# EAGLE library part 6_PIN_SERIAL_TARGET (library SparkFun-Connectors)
6-pin header connection for use with the "FTDI BASIC" pinout - TARGET SIDE. Also known as "Arduino Serial Program Header". It is used to mate with our FTDI Basic serial programmers using the Arduino IDE. Note, this device has "TARGET" in the name. It is intended to be used on a design that contains a target micro-controller that you wish to program. The "sister" device, named "CABLE" is inteneded to be used on a design that usually lives on the end of your USB cable and prvides the converter chip (FTDI232 or FTDI231x) to commnicate serial RX/TX. You can populate with some of these: Break Away Headers - Straight (PRT-00116) For reference (or to suit your programming needs) check out these designs: SparkFun FTDI Basic Breakout - 5V (DEV-09716) SparkFun FTDI Basic Breakout - 3.3V (DEV-09873) SparkFun FTDI SmartBasic (DEV-12935) SparkFun Beefy 3 - FTDI Basic Breakout (DEV-13746)
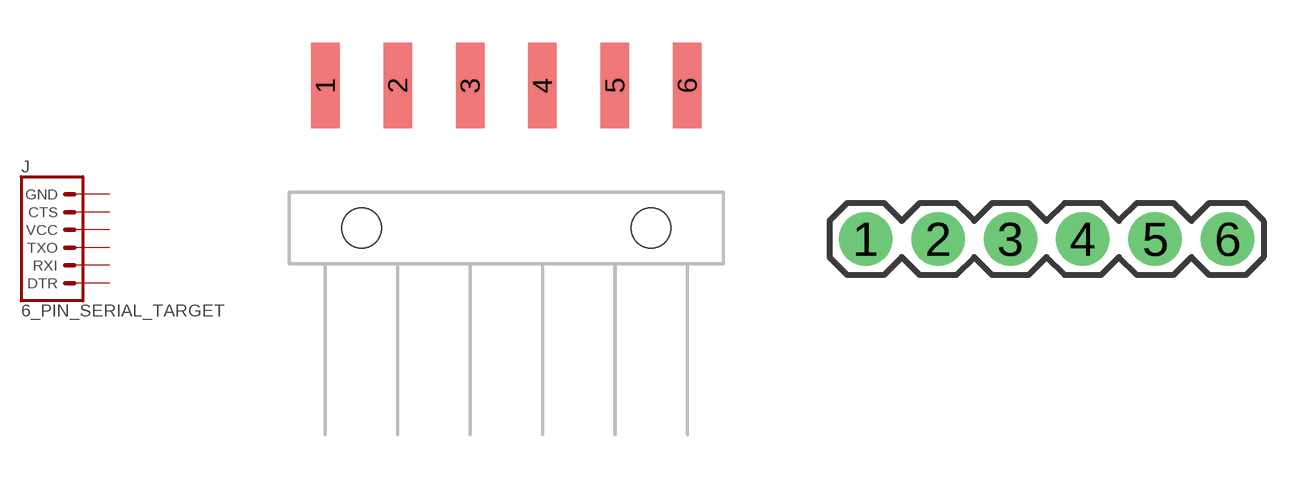
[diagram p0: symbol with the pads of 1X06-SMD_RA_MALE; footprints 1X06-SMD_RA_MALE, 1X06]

Designator prefix J

## 6_PIN_SERIAL_TARGETSMD (PROD_ID: CONN-08971)  [1X06-SMD_RA_MALE]
1  DTR  pas
2  RXI  pas
3  TXO  pas
4  VCC  pas
5  CTS  pas
6  GND  pas

## 6_PIN_SERIAL_TARGET_SILK  [1X06]
Pads as for 1X06-SMD_RA_MALE

## 6_PIN_SERIAL_TARGETRA_LOCK  [MOLEX_1X6_RA_LOCK]
1  GND  pas
2  CTS  pas
3  VCC  pas
4  TXO  pas
5  RXI  pas
6  DTR  pas

## 6_PIN_SERIAL_TARGETLONGPADS  [1X06_LONGPADS]
Pads as for 1X06-SMD_RA_MALE

## 6_PIN_SERIAL_TARGETLOCK (PROD_ID: CONN-08437)  [1X06_LOCK]
Pads as for 1X06-SMD_RA_MALE

## 6_PIN_SERIAL_TARGETPTH-KIT  [1X06-KIT]
Pads as for 1X06-SMD_RA_MALE

## 6_PIN_SERIAL_TARGETSILK  [6_PIN_SERIAL_TARGET_SIDE_W_SILK]
P$1  DTR  pas
P$2  TXO  pas
P$3  RXI  pas
P$4  VCC  pas
P$5  CTS  pas
P$6  GND  pas

## 6_PIN_SERIAL_TARGETRA_SMT (PROD_ID: CONN-08971)  [6_PIN_SERIAL_TARGET_SIDE_RA_SMT]
1  DTR  pas
2  TXO  pas
3  RXI  pas
4  VCC  pas
5  CTS  pas
6  GND  pas

## 6_PIN_SERIAL_TARGET_NO_SILK  [1X06_NO_SILK]
Pads as for 1X06-SMD_RA_MALE

## 6_PIN_SERIAL_TARGETVERT_SMT (PROD_ID: CONN-10203)  [6_PIN_SERIAL_TARGET_SIDE_VERT_SMT]
1  DTR  pas
1-2  DTR  pas
2  TXO  pas
2-2  TXO  pas
3  RXI  pas
3-2  RXI  pas
4  VCC  pas
4-2  VCC  pas
5  CTS  pas
5-2  CTS  pas
6  GND  pas
6-2  GND  pas

## Footprint 1X06-SMD_RA_MALE (pad centres in mm)
SMD - 6 Pin Right Angle Male Header tDocu layer shows pin locations. Specifications: Pin count:6 Pin pitch:0.1" Example device(s): CONN_06
smd 1 x 3: 1 -6.35,5; 2 -3.81,5; 3 -1.27,5; 4 1.27,5; 5 3.81,5; 6 6.35,5
hole 1.4 at -5.08,0
hole 1.4 at 5.08,0

## Footprint 1X06 (pad centres in mm)
Plated Through Hole - 6 Pin Specifications: Pin count:6 Pin pitch:0.1" Example device(s): CONN_06
drill 1.016 pad 1.88: 1 0,0; 2 2.54,0; 3 5.08,0; 4 7.62,0; 5 10.16,0; 6 12.7,0

## Footprint MOLEX_1X6_RA_LOCK (pad centres in mm)
Molex 6-Pin Plated Through-Hole Right Angle Locking Footprint Holes are offset 0.005" from center to hold pins in place during soldering. tPlace shows location of connector. Specifications: Pin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
drill 1.016 pad 1.88: 1 0,0.127; 2 2.54,-0.127; 3 5.08,0.127; 4 7.62,-0.127; 5 10.16,0.127; 6 12.7,-0.127

## Footprint 1X06_LONGPADS (pad centres in mm)
Plated Through Hole - 6 Pin with Long Pads Specifications: Pin count:6 Pin pitch:0.1" Example device(s): CONN_06
drill 1.118 pad 1.88 long: 1 0,0; 2 2.54,0; 3 5.08,0; 4 7.62,0; 5 10.16,0; 6 12.7,0

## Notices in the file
Licensing: Creative Commons ShareAlike 4.0 International - https://creativecommons.org/licenses/by-sa/4.0
